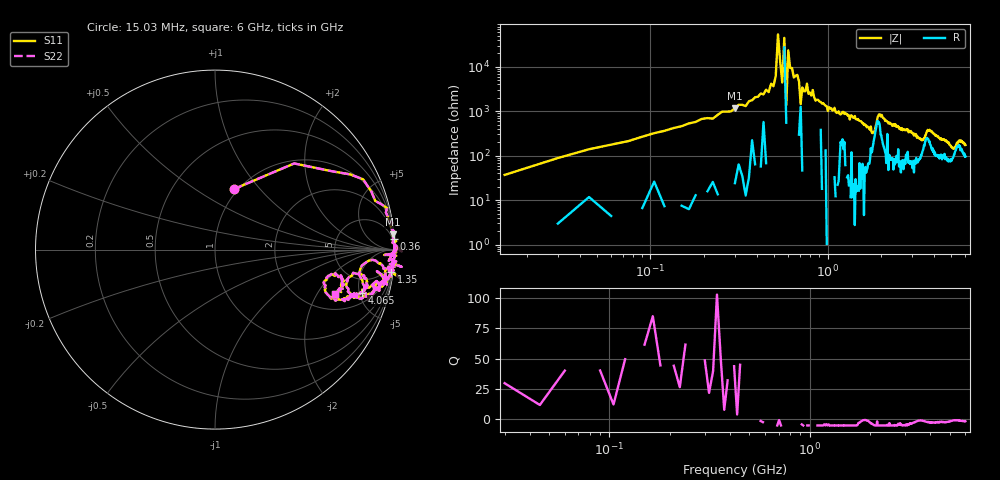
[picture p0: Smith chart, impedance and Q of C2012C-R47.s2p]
!	Network	Analyzer	HP8753E.07.74:	Oct	30	2002	Serial	No.	JP38451487
!	Hewlett-Packard
!	28	Aug	2009	12:02:15
!	Frequency	S11	S21	S12	S22
#	HZ	S	RI	R	50
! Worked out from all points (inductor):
!   400 points, 15.03 MHz to 6 GHz, reference 50 ohm
!   read as one part in series: L = 461 nH near 45.03 MHz
!   highest Q = 48.5 at 300 MHz (marker M1), where L = 619 nH
!   self-resonance near 450 MHz
!   S11 on the Smith chart (normalised r, x): 15.03 MHz: 0.96, +0.74; 360 MHz: 2, +33; 1.35 GHz: 1, -16; 4.065 GHz: 2.96, -5.30; 6 GHz: 2.90, -2.92
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1.502992e7  0.105 0.337  0.895 -0.337  0.895 -0.337  0.105 0.337
7.502962e7  0.825 0.392  0.175 -0.392  0.175 -0.392  0.825 0.392
3.000285e8  0.991 0.0847  0.009 -0.0847  0.009 -0.0847  0.991 0.0847
3.600282e8  0.995 0.0593  0.0047 -0.0593  0.0047 -0.0593  0.995 0.0593
4.950275e8  1 0.0271  -0.00347 -0.0271  -0.00347 -0.0271  1 0.0271
5.100274e8  0.999 0.0161  0.0011 -0.0161  0.0011 -0.0161  0.999 0.0161
5.250274e8  1 0.000427  -0.00183 -0.000427  -0.00183 -0.000427  1 0.000427
5.550272e8  1 0.0225  -0.00305 -0.0225  -0.00305 -0.0225  1 0.0225
5.700272e8  0.999 -0.00177  0.00137 0.00177  0.00137 0.00177  0.999 -0.00177
5.850271e8  0.968 -0.0627  0.0323 0.0627  0.0323 0.0627  0.968 -0.0627
6.00027e8  1 -0.00403  -0.0014 0.00403  -0.0014 0.00403  1 -0.00403
7.050265e8  0.942 -0.03  0.0579 0.03  0.0579 0.03  0.942 -0.03
7.650262e8  0.995 -0.0233  0.0054 0.0233  0.0054 0.0233  0.995 -0.0233
1.020025e9  0.995 -0.0808  0.00504 0.0808  0.00504 0.0808  0.995 -0.0808
1.350023e9  0.983 -0.124  0.0175 0.124  0.0175 0.124  0.983 -0.124
1.785021e9  0.838 -0.214  0.162 0.214  0.162 0.214  0.838 -0.214
2.01002e9  0.947 -0.104  0.0534 0.104  0.0534 0.104  0.947 -0.104
3.015015e9  0.878 -0.255  0.122 0.255  0.122 0.255  0.878 -0.255
4.00501e9  0.833 -0.23  0.167 0.23  0.167 0.23  0.833 -0.23
4.06501e9  0.819 -0.242  0.181 0.242  0.181 0.242  0.819 -0.242
5.010005e9  0.649 -0.266  0.351 0.266  0.351 0.266  0.649 -0.266
6e9  0.671 -0.246  0.329 0.246  0.329 0.246  0.671 -0.246
